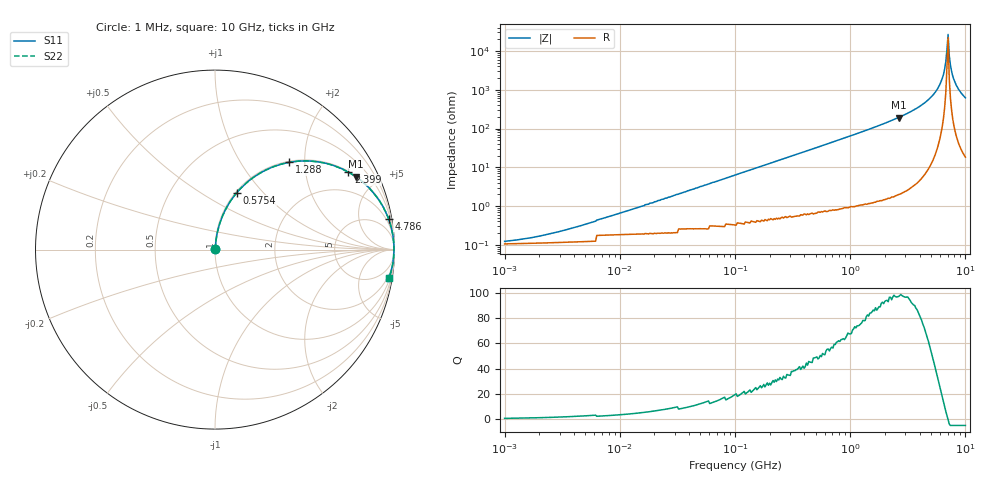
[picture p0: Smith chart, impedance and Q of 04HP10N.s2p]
# MHz S MA R 50
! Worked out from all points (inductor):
!   401 points, 1 MHz to 10 GHz, reference 50 ohm
!   read as one part in series: L = 10 nH near 5.888 MHz
!   highest Q = 97.1 at 2.63 GHz (marker M1), where L = 11.6 nH
!   self-resonance near 6.918 GHz
!   S11 on the Smith chart (normalised r, x): 1 MHz: 1.00, +0.00; 575.4 MHz: 1.01, +0.73; 1.288 GHz: 1.02, +1.67; 2.399 GHz: 1.03, +3.41; 4.786 GHz: 1, +11; 10 GHz: 1, -12
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1  0.001271 29.5  0.999 -0.0  0.999 -0.0  0.001271 29.5
2.042  0.001766 46.4  0.999 -0.1  0.999 -0.1  0.001766 46.4
4.677  0.003253 64.3  0.999 -0.2  0.999 -0.2  0.003253 64.3
21.878  0.014 80.7  0.998 -0.8  0.998 -0.8  0.014 80.7
102.329  0.064 83.3  0.995 -3.7  0.995 -3.7  0.064 83.3
467.735  0.282 72.4  0.953 -16.3  0.953 -16.3  0.282 72.4
575.44  0.34 69.0  0.934 -19.9  0.934 -19.9  0.34 69.0
1288.25  0.638 49.6  0.762 -39.6  0.762 -39.6  0.638 49.6
2187.762  0.832 33.1  0.547 -56.3  0.547 -56.3  0.832 33.1
2398.833  0.859 30.2  0.504 -59.2  0.504 -59.2  0.859 30.2
2630.268  0.883 27.4  0.46 -62.0  0.46 -62.0  0.883 27.4
3715.352  0.952 17.1  0.295 -72.2  0.295 -72.2  0.952 17.1
4786.301  0.982 10.1  0.176 -78.9  0.176 -78.9  0.982 10.1
6025.596  0.995 4.1  0.071 -83.6  0.071 -83.6  0.995 4.1
6456.542  0.996 2.3  0.04 -83.5  0.04 -83.5  0.996 2.3
6760.83  0.997 1.1  0.019 -79.7  0.019 -79.7  0.997 1.1
7079.458  0.997 -0.1  0.003737 32.7  0.003737 32.7  0.997 -0.1
7244.36  0.997 -0.7  0.013 74.8  0.013 74.8  0.997 -0.7
7585.776  0.996 -1.9  0.033 82.3  0.033 82.3  0.996 -1.9
8128.305  0.994 -3.7  0.064 83.1  0.064 83.1  0.994 -3.7
8912.509  0.99 -6.1  0.106 81.8  0.106 81.8  0.99 -6.1
10000  0.983 -9.1  0.159 79.2  0.159 79.2  0.983 -9.1
